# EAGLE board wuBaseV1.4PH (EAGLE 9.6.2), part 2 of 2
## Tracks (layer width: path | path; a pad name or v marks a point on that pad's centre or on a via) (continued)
GND  (via drill 0.35, 0.5) (continued)
  Bottom 0.508: R108.2 77.28,29.32 78.26,28.34 79,28.34 v79.86,29.2 | v90.8,32.74 90.36,32.29 89.83,32.29 89.64,32.48 C108.2 | v84.13,18.95 83.82,18.64 C66.2 | v83.31,17.47 83.31,17.7 83.3,17.71 C66.2 | C67.2 82.25,20.04 83.3,18.98 C66.2 | C59.2 77.03,16.99 77.16,17.12 v77.29,17.12 | C35.2 98.76,25.37 v98.5,25.62 | C119.2 87.34,23.29 88.28,24.23 v89.05,24.23 | 91.9,18.77 91.95,18.82 J1.1 | 105.1,25.62 C111.1 105.24,26.02 106,26.77 106.5,26.77 | 104.34,26.52 v104.34,27.78 | 101.7,23.47 102.05,23.81 | v92.84,17.39 92.76,17.39 | 103.33,24.1 C50.2 103.2,24.36 102.3,24.36 C51.2 | 102.39,23.76 102.44,23.81 | v103.4,22.83 103.45,22.78 104.78,22.78 v104.83,22.83 | C49.2 50.79,34.37 v52.53,33.24
  Bottom 0.61: C130.2 88.39,24.75 88.92,24.23 v89.05,24.23 | 91.9,18.77 91.01,18.77 v90.73,18.49 | v93.19,28.32 93.19,27.55 91.69,26.06 91.69,24.05 92.46,23.29 92.46,22.18 | 92.46,22.18 92.46,21.49 91.95,20.98 J1.1 91.95,18.21 92.76,17.39 | C50.2 103.97,24.49 105.1,25.62 | 101.83,23.47 100.89,22.53 v100.46,22.96 100.46,22.43 98.67,22.43 | C51.2 102.05,23.81 102.44,23.81 103.04,23.81 | J1.4 93.22,17.02 v92.84,17.39 | v104.83,22.83 105.24,23.25 C111.1 | 103.04,23.81 102.72,23.5 103.33,22.89 103.33,24.1 103.04,23.81 | 102.39,23.76 v102.39,22.86 102.39,22.98 101.91,23.47 101.83,23.47 | 101.83,23.47 101.7,23.47 | C3.1 v36.82,19.26 | C37.1 40.26,15.96 | 92.46,22.18 97.14,22.18
  Bottom 0.813: C111.1 104.34,26.52 | C21.1 37.45,19.77 37.07,21.16 36.44,21.8 v34.28,22.18
  Bottom 1.016: v36.82,19.26 37.45,19.77
  Bottom 1.27: 37.45,19.77 38.11,19.13 | 44.8,11.99 v45.09,10.79 v43.92,10.89 42.62,12.54
  Bottom 1.524: 38.11,19.13 40.26,15.96 42.62,12.54 44.8,11.99
  other vias: 83.2,28.67 85.11,28.67 87.02,28.67 85.11,30.2 85.11,27.28 72.34,33.88 110.08,25.65 90.27,34.52 78.44,32.48 79.71,32.48 80.98,32.48 79.83,23.47 78.82,23.21 101.55,27.78 102.95,26.39 80.67,24.33 98.96,31.34 107.64,33.88 53.92,33.75 71.7,34.64 80.21,16.99 87.83,12.92 109.57,20.19 73.74,12.92 91.67,21.33
  pour Bottom (isolate 0.203): 70.73,31.25 76.83,31.25 76.83,23.58 71.11,23.58 71.11,22.43 72.25,21.29 78.86,21.29 78.86,17.48 73.4,17.48 71.21,15.32 71.21,11.49 74.28,10.98 108.22,10.98 111.19,13.95 111.19,32.92 108.14,35.95 74.23,35.95 70.73,35.31
  pour Route2: 71.21,14.84 59.91,14.84 56.86,14.07 47.58,12.67 44.15,13.05 42.88,13.69 40.72,18.26 36.82,22.05 35.17,22.43 35.17,25.86 34.79,26.75 32.88,27.13 31.61,30.18 30.34,30.18 30.34,27.64 30.85,27.64 33.39,25.1 33.39,21.8 30.85,19.26 27.55,19.26 25.01,21.8 25.01,25.1 26.63,26.7 25.01,28.35 23.36,26.75 23.36,21.67 24.12,19.77 25.64,18.24 27.68,17.23 30.85,16.34 38.22,16.34 42.03,11.13 44.15,9.6 59.21,13.26 61.27,13.18 71.21,11.49
  pour Route2: 69.43,23.58 76.83,23.58 76.83,31.25 70.73,31.25 70.73,33.36 64.76,33.36 59.3,32.47 53.08,32.47 52.06,33.1 52.06,34.12 54.47,34.75 59.3,33.61 61.2,33.61 74.26,35.95 108.19,35.95 111.19,32.92 111.19,13.95 108.22,10.98 74.23,10.98 71.21,11.49 71.21,19.77 69.43,22.7
  pour Route15: 48.21,35.15 48.21,33.88 48.5,33.61 51.51,33.5 52.53,32.74 52.78,33.75 51.55,34.5 49.27,35.39 48.46,35.4
  cutout Bottom: 94.95,33.24 96.72,33.24 96.72,32.1 94.95,32.1
  pour Route15 (no thermals): 30.85,19.26 27.55,19.26 25.01,21.8 25.01,25.1 26.63,26.7 23.23,30.05 22.6,29.93 20.95,28.4 19.93,26.24 19.93,22.56 20.31,21.93 20.82,21.67 21.2,21.67 21.2,26.12 21.45,26.12 21.45,21.67 21.71,21.67 21.71,26.24 21.96,26.24 21.96,21.67 22.21,21.67 22.21,26.24 22.47,26.24 22.47,21.67 22.72,21.67 22.72,26.24 22.98,26.24 22.98,21.67 23.23,21.67 23.23,26.12 23.48,26.12 23.48,21.42 24.12,19.77 25.64,18.24 27.68,17.23 30.85,16.34 34.79,16.34 37.68,18.4 39.23,20.66 39.23,22.59 39.87,23.83 39.87,24.21 39.49,24.59 37.02,25.23 36.57,25.74 35.93,29.8 35.68,31.83 35.68,32.59 35.55,32.98 35.3,33.23 33.9,33.74 32.63,34.5 31.23,34.88 26.02,34.88 25.39,34.5 25.39,34.37 30.98,34.37 30.98,34.12 25.06,34.12 24.88,33.74 24.88,31.58 26.15,31.58 26.15,32.21 25.26,32.21 25.26,32.47 26.15,32.47 26.15,33.23 25.39,33.23 25.39,33.48 31.87,33.48 31.87,33.23 30.22,33.23 30.22,32.47 32.25,32.47 32.25,32.21 30.85,32.21 30.85,31.58 32.25,31.58 32.25,31.32 30.85,31.32 30.85,30.69 32.25,30.69 32.25,30.43 30.22,30.43 30.22,29.67 31.87,29.67 31.87,29.42 25.39,29.42 25.39,29.67 26.15,29.67 26.15,30.43 25.26,30.43 25.26,30.69 26.15,30.69 26.15,31.32 24.88,31.32 24.88,29.04 25.14,28.78 30.22,28.78 30.22,28.53 25.39,28.53 26.28,27.64 30.85,27.64 33.39,25.1 33.39,21.8
  pour Top: 64.76,33.36 72.63,33.36 72.63,35.64 61.2,33.61 59.3,33.61 54.47,34.75 52.06,34.12 52.06,33.1 53.08,32.47 59.3,32.47
  cutout Bottom: 88,23.45 88,21.93 88.64,21.93 88.64,23.45
  cutout Bottom: 69.84,26.88 70.47,26.88 70.47,25.86 69.84,25.86 69.84,26.75
HVMON_A
  Bottom 0.305: R32.1 R31.2 C36.1
HVMON_B  (via drill 0.35)
  Top 0.203: v56.59,19.66 56.08,19.66 55.32,20.29 v54.69,21.69 | v95.84,24.23 94.69,24.23 93.42,22.96 91.36,22.96 90.42,22.02 87.4,22.02 v86.84,21.46
  Route15 0.203: v56.59,19.66 56.72,19.78 63.07,19.78 64.34,21.05 69.55,21.05 69.78,21.28 86.67,21.28 v86.84,21.46
  Bottom 0.203: v95.84,24.23 96.27,24.66 99.95,24.66 100.17,24.88 C35.1 100.17,25.95 101.37,27.15 101.93,27.15 R30.2
  Bottom 0.254: R31.1 54.47,22.43 v54.69,21.69
K
  Top 0.508: R29.2 35.42,5.92 K.P$1
  Bottom 0.508: C48.2 34.03,8.59 K.P$1
  pour Route15 (no thermals): 32.38,9.73 33.14,10.24 34.15,10.11 35.55,9.35 36.69,7.45 36.82,6.43 35.68,4.91 35.04,4.91 33.14,7.96 32.38,8.21
K-DY1-AA  (via drill 0.35)
  Top 0.305: D14.2 v29.84,6.56 | R28.1 v29.84,6.56 | D13.1 v29.84,6.56
  Bottom 0.305: R14.2 C32.2 v29.84,6.56 C33.1 R15.1
  pour Route15: 27.47,5.52 28.44,6.2 28.49,7.35 30.9,7.73 31.36,7.07 31.33,5.67 32.02,5.21 32.1,5.01 32.1,4.15 31.61,1.94 30.72,0.97 27.68,0.97 26.91,1.35 26.71,2.01 26.71,3.28 27.45,4.45
K-DY1-AB  (via drill 0.35)
  Top 0.305: v29.84,9.1 R28.2
  Bottom 0.305: C47.2 v29.84,9.1 C48.1
  pour Route15: 28.18,9.23 28.18,7.96 28.34,7.78 31.28,8.16 31.54,8.36 31.51,9.76 31.08,10.14 28.59,9.81
K-DY1-BA  (via drill 0.35)
  Top 0.305: D12.1 v25.39,6.69 | D13.2 v25.39,6.69 | R27.1 v25.39,6.69
  Bottom 0.305: C31.2 R13.2 v25.39,6.69 C32.1 R14.1
  pour Route15: 27.17,7.45 25.26,7.83 23.74,9.1 23.36,9.1 23.1,8.84 23.1,7.7 22.34,7.09 22.09,6.71 22.09,5.92 22.37,5.04 22.37,3.64 22.6,2.24 23.61,1.22 24.88,1.1 25.64,1.35 25.85,1.86 25.85,3.51 26.66,4.65 26.66,5.67 27.42,6.3 27.42,7.07
K-DY1-BB  (via drill 0.35)
  Top 0.305: v26.02,9.23 R27.2
  Bottom 0.305: C46.2 v26.02,9.23 C47.1
  pour Route15: 22.49,9.63 22.47,10.75 22.85,11.13 23.87,10.88 25.39,10.11 26.79,9.86 27.17,9.61 27.42,9.23 27.42,8.21 27.17,7.96 25.39,8.21 23.74,9.48 23.26,9.38 22.85,9.35
KA  (via drill 0.35)
  Top 0.305: D14.1 v34.15,4.53 R29.1
  Bottom 0.305: v34.15,4.53 R15.2 C33.2
  pour Route15 (no thermals): 32.17,6.3 32.3,5.95 33.01,5.54 33.01,3.13 33.26,2.88 33.77,2.88 34.28,3.26 34.79,4.53 32.88,7.57 32.38,7.57 32.17,7.07
N$11
  Bottom 0.254: IC7.2 60.41,22.58 60.15,22.31 C79.2 59.77,22.2 R78.2
N$15
  Bottom 0.254: IC7.3 60.41,23.08 60.15,23.35 C83.1 59.77,23.47 R84.2
N$16
  Bottom 0.203: R87.2 56.88,24.23
  Bottom 0.254: R86.1 R84.1 57.77,23.34 56.88,23.34 | 56.88,23.34 C81.2 56.08,23.33 R83.2 | 56.88,24.23 56.88,23.34
N$17
  Bottom 0.254: R71.1 R78.1 57.77,22.32 56.88,22.32 | C81.1 56.88,22.32 | R77.2 56.85,22.29 56.88,22.32
N$18
  Bottom 0.254: IC7.1 60.42,21.34 C79.1 59.64,21.31 59.25,20.93 R71.2
N$19
  Bottom 0.254: IC7.4 60.39,24.35 C83.2 59.64,24.35 59.25,24.74 R86.2
N$22
  Bottom 0.203: R79.1 65.74,24.65 65.74,23.59 64.72,22.58
  Bottom 0.254: IC7.11 64.72,22.58
N$23
  Bottom 0.203: R85.1 65.23,26.68 65.23,23.84 64.47,23.08
  Bottom 0.254: IC7.10 64.47,23.08
N$25
  Bottom 0.254: IC6.2 58.61,28.66 C75.2 57.35,28.67 56.46,28.67 R69.2
N$26
  Bottom 0.254: IC6.3 58.05,29.18 57.66,29.57 57.48,29.57 C80.1 57.21,29.84 56.56,29.84 R73.2
N$27
  Bottom 0.254: R67.1 R69.1 55.23,28.93 54.34,28.93 C76.1 R68.2
N$28
  Bottom 0.254: R81.1 R73.1 55.23,29.94 54.34,29.94 C76.2 R72.2 53.8,30.84 53.43,31.2 R80.2
N$29
  Bottom 0.254: IC6.1 58.37,28.18 57.86,27.66 C75.1 57.18,27.66 57.12,27.59 57.06,27.53 R67.2
N$30
  Bottom 0.254: IC6.4 58.34,29.68 58.24,29.78 58.24,30.18 57.73,30.7 C80.2 57.06,30.7 56.45,31.34 R81.2
N$33
  Bottom 0.254: IC6.11 62.44,28.68 62.56,28.8 R70.1
N$34
  Bottom 0.254: IC6.10 61.92,29.18 62.7,29.95 R74.1
NRST
  Top 0.254: IC8.7 107.14,28.03 107.7,27.48 C94.1
REFH  (via drill 0.35)
  Top 0.254: IC10.9 67.21,27.15 66.66,26.61 | 66.66,26.61 C98.2 66.59,26.64 C101.1 | IC10.7 67.91,28.15 v67.77,28.29 | v67.26,25.88 67.26,26.01 66.66,26.61
  Route15 0.254: v67.77,28.29 67.13,27.66 67.13,26.01 v67.26,25.88
REFL  (via drill 0.35)
  Top 0.254: IC10.8 67.17,27.65 C98.1 | IC10.10 67.91,26.65 v67.77,26.51 | v67.26,28.93 66.62,28.29 C98.1 | C97.1 66.46,28.04 C98.1
  Route2 0.254: v67.77,26.51 67.13,27.15 67.13,28.8 v67.26,28.93
SPI1_MISO  (via drill 0.35)
  Top 0.203: IC8.32 99.49,27.01 98.31,27.01 v98.22,26.92 | v71.09,32.94 70.72,32.57 IC10.61 | v93.8,25.27 93.8,24.99 93.12,24.3 90.68,24.3 89.61,23.24 86.28,23.24 84.99,21.94 v83.9,21.94
  Route15 0.203: v73.48,21.81 73.66,21.64 83.59,21.64 v83.9,21.94 | v72.47,22.17 v72.47,22.18 72.47,29.18 71.09,30.55 v71.09,32.94
  Bottom 0.203: v73.48,21.81 73.38,21.71 72.83,21.71 72.47,22.07 v72.47,22.17 | v98.22,26.92 95.07,26.92 94.45,26.29 R89.2 93.83,25.24 v93.8,25.27
SPI1_MOSI
  Top 0.203: IC8.33 98.88,26.53 98.75,26.41 96.11,26.41 95.07,25.37 94.77,25.37 93.24,23.85 90.87,23.85 89.84,22.81 86.6,22.81 84.92,21.13 72.78,21.13 71.72,22.18 IC10.22
SPI1_SCK
  Top 0.203: IC8.39 101.2,23.75 101.04,23.59 99.9,23.59 99.19,24.3 96.52,24.3 96.09,24.74 94.69,24.74 93.37,23.41 91.14,23.41 90.1,22.38 86.93,22.38 85.3,20.75 72.42,20.75 71.22,21.94 IC10.21
SPI2_MISO
  Top 0.152: IC9.14 89.39,26.42 89.68,26.13 93.5,26.13 96.9,29.53 IC8.27
SPI2_MOSI  (via drill 0.35)
  Top 0.152: IC9.17 89.67,27.92 90.32,27.28 93.04,27.28 94.82,29.05 v94.82,29.31
  Top 0.203: IC8.28 v97.08,29.03
  Bottom 0.152: v94.82,29.31 95.2,28.93 96.98,28.93 v97.08,29.03
SPI2_SCK
  Top 0.152: IC9.15 89.53,26.92 89.94,26.51 93.37,26.51 96.89,30.03 IC8.26
SYNC  (via drill 0.35)
  Top 0.203: v93.16,29.18 92.9,28.92 IC9.19
  Route15 0.203: v93.16,29.18 92.91,28.93 92.35,28.93 91.05,27.63 91.05,19.08 91.39,18.74 91.39,18.26 90.88,17.75 v90.88,16.68
  Bottom 0.203: J1.8 95.76,14.63 95.19,14.07 91.39,14.07 91.01,14.45 91.01,16.56 v90.88,16.68
TIM2_CH3
  Top 0.203: IC8.12 106.72,30.53 107.02,30.83 107.02,31.09 107.53,31.59 R92.2
TIM2_CH3_SOFT  (via drill 0.35)
  Top 0.203: v46.28,11.76 49.01,11.51 59.97,14.05 70.6,14.05 72,12.65 v72.38,12.65 | v109.84,24.59 109.46,24.97 109.46,28.4 109.59,28.53 109.58,31.31 109.3,31.59 R92.1
  Top 0.305: IC1.3 36.2,19.91 v36.44,20.15
  Route15 0.203: v46.28,11.76 45.39,11.96 42.67,12.52 37.58,19.89 v36.44,20.15 | v72.38,12.65 72.96,12.07 104.82,12.07 108.32,15.58 108.32,20.4 109.84,21.93 v109.84,24.59
TRIGOUT  (via drill 0.35)
  Top 0.203: IC8.15 104.7,32.26 v104.6,32.36
  Top 0.254: v96.22,17.75 96.22,17.6 96.03,17.41 IC13.1 | v94.54,17.75 94.54,17.6 94.73,17.41 IC13.3
  Route15 0.152: v104.6,32.36 104.6,29.94 104.34,29.69 99.9,29.69 98.93,28.72 98.43,28.72 96.88,27.17 96.88,24.73 v97.83,23.78 | v94.54,17.75 94.54,17.98 95.07,18.51 95.84,18.51 96.22,18.13 v96.22,17.75
  Bottom 0.152: v97.83,23.78 97.73,23.68 97.73,21.8 97.22,21.29 96.64,21.29 96.38,21.04 96.38,17.92 v96.22,17.75
TRIGOUT_N  (via drill 0.35)
  Top 0.203: v93.83,18 93.8,18 93.45,17.65 93.45,16.89 93.11,16.55 R33.1
  Bottom 0.254: J1.5 94.31,19.54 94.31,18.49 v93.83,18
TRIGOUT_NA
  Top 0.203: IC13.4 93.42,14.81 R33.2 C123.1
TRIGOUT_P  (via drill 0.35)
  Top 0.203: R34.1 98.14,17 v98.5,17.37
  Route15 0.152: v94.03,17.17 94.11,17.24 98.38,17.24 v98.5,17.37
  Bottom 0.254: J1.6 94.41,15.73 94.41,16.79 v94.03,17.17
TRIGOUT_PA
  Top 0.203: R34.2 97.14,15.03 C124.1 96.2,14.98 IC13.6
TVS_OUT
  Top 0.305: R2.2 D1.C
UART_RXD_P  (via drill 0.35)
  Route15 0.152: v98.05,27.61 97.23,26.79 97.23,25.29 98.53,24 v98.53,23.8
  Bottom 0.152: 97.66,17.32 97.66,21.16 98.02,21.51 98.02,23.29 v98.53,23.8
  Bottom 0.203: R90.1 98.85,28.41 v98.05,27.61
  Bottom 0.254: 97.66,17.32 98.3,16.68 J1.12
UART_TXD_A  (via drill 0.35)
  Top 0.152: 105.63,21.16 105.63,21.32 105.4,21.54 104.64,21.54 104.08,20.99 104.08,20.92 | 105.63,21.16 IC11.1 | R93.1 105.64,21.16 105.63,21.16 | 104.08,20.92 104.33,20.67 IC11.3 | v96.77,22.95 97.08,22.64 98.16,22.64 101.84,21.54 103.46,21.54 104.08,20.92
  Top 0.203: R91.1 97.01,27.02 95.96,27.02 v95.33,26.39
  Route15 0.152: v96.77,22.95 96.77,22.98 96.26,23.48 95.84,23.48 95.33,24 v95.33,26.39
UART_TXD_N  (via drill 0.35)
  Top 0.203: v101.12,18.11 101.76,18.11 R99.1
  Bottom 0.254: J1.15 100.84,18.39 v101.12,18.11
UART_TXD_NA
  Top 0.203: IC11.4 102.95,17.92 R99.2 C112.1
UART_TXD_P  (via drill 0.35)
  Top 0.203: R98.1 100.08,16.95 v100.08,17.45
  Bottom 0.254: J1.14 99.57,16.81 100.08,17.32 v100.08,17.45
UART_TXD_PA  (via drill 0.35)
  Top 0.203: v103.02,15.77 102.84,15.59 102.43,15.59 R98.2 | IC11.6 105.73,17.81 v106.36,17.81 107.18,17.81 C113.1
  Route15 0.203: v103.02,15.77 105.06,17.8 v106.35,17.8 v106.36,17.81
USART1_RX  (via drill 0.35)
  Top 0.152: IC8.31 98.76,27.53 v98.73,27.55
  Bottom 0.203: R90.2 98.88,27.41 v98.73,27.55
USART1_TX
  Top 0.152: IC8.30 98.89,28.03 98.76,28.16 97.19,28.16 R91.2
VCCPLL  (via drill 0.5)
  Top 0.203: IC9.29 85.86,32.47 86.13,32.74 86.13,33.17 v86.23,33.27
  Top 0.508: v90.8,33.7 90.86,33.64 91.8,33.64 C109.1
  Bottom 0.508: v86.23,33.27 86.64,32.86 R94.2 87.67,32.86 C108.1 88.04,33 88.31,33.27 90.06,33.27 90.5,33.7 v90.8,33.7
VDD_AMP  (via drill 0.5)
  Top 0.305: L17.1 69.41,19.78 L16.1 72.24,19.27 73.14,18.37 74.79,18.37 76.04,19.61 88.41,19.61 89.87,18.16
  Top 0.508: v97.03,18.03 97.03,18.72 C115.1 92.44,18.75 91.3,17.61 90.41,17.61 89.87,18.16
  Bottom 0.508: J1.9 v97.03,18.03
VDDA-ADC  (via drill 0.5)
  Top 0.203: IC10.17 69.22,22.89 69.04,22.7
  Top 0.254: IC10.63 69.72,32.12 69.59,32.25 | IC10.64 69.22,32.17 69.14,32.25 | 68.38,32.25 v68.28,32.36 | IC10.1 68.21,31.15 68.1,31.26 | IC10.16 68.41,23.65 68.29,23.53 68.21,23.53
  Top 0.508: 68.21,23.53 v67.66,22.98 67.78,22.98 68.06,22.7 69.04,22.7 | 68.38,32.25 69.14,32.25 69.59,32.25 | 68.1,31.26 68.1,32.18 v68.28,32.36
  Bottom 0.406: v68.28,32.36 68.54,32.09 C91.1 68.54,30.06 69.38,29.22 C128.2 69.55,26.21 L18.2 69.55,24.58 68.78,23.81 C103.1
  Bottom 0.508: v67.66,22.98 68.27,23.59 C103.1
VDDFPGA  (via drill 0.5)
  Top 0.508: C114.1 97.97,21.4 97.93,21.36 v95.71,21.36 95.71,20.93 L19.1
  Bottom 0.508: v95.71,21.36 95.76,21.31 J1.7
VDDFPGA-FILT  (via drill 0.5)
  Top 0.203: v84.36,24.24 v84.35,24.23 | IC9.30 85.36,32.87 v85.31,32.91
  Top 0.229: IC9.5 v84.36,24.24
  Top 0.508: L19.2 93.81,20.16 93.1,19.45 90.5,19.45 v90.37,19.33
  Route15 0.406: v84.35,24.23 85.62,24.23 86.39,23.47 88.6,23.47 90.37,21.69 v90.37,19.33
  Route15 0.61: v91.46,31.21 91.08,31.21 89.81,32.48 88.82,32.48 88.61,32.28 85.95,32.28 v85.31,32.91
  Bottom 0.508: C107.1 85.11,32.71 v85.31,32.91 86.37,31.86 R94.1
  Bottom 0.61: v91.46,31.21 91.59,31.09 91.59,29.31 88.63,26.36 C130.1 87.29,26.36 85.55,24.61 C100.1 84.73,24.61 v84.35,24.23
VDDSW  (via drill 0.5)
  Top 0.508: C122.1 96.97,12.8 v95.94,12.8
  Route15 0.508: v94.56,33.88 97.11,33.88 97.87,34.64 108.15,34.64 109.98,32.81 109.98,26.95 109.04,26.01 109.04,22.32 v108.53,21.81
  Bottom 0.406: IC12.4 94.66,33.79 v94.56,33.88 94.56,32.48 94.32,32.24 | C132.2 R101.2 94.32,32.24 | 94.32,32.24 94.53,32.24 IC12.3
  Bottom 0.508: J1.10 97.03,13.61 96.22,12.8 v95.94,12.8 104.65,12.8 107.69,15.83 107.69,20.91 108.53,21.76 v108.53,21.81
VDDSW-FILT  (via drill 0.35, 0.5)
  Top 0.305: v45.92,12.37 49.12,12.09 59.97,14.45 75.19,14.45 76.95,16.21 82.03,16.21 v82.54,16.72
  Top 0.508: v92.41,29.69 92.41,29.75 93.42,30.77 L13.2
  Route15 0.305: v89.36,21.05 88.8,20.49 84.58,20.49 82.54,18.46 v82.54,16.72 | v45.92,12.37 45.42,12.37 42.95,12.87 37.81,20.45 v35.8,20.91
  Bottom 0.406: C119.1 89.36,22.69 v89.36,21.05 | v35.8,20.91 35.41,20.91 R1.1
  Bottom 0.508: C119.1 90.25,23.61 90.25,26.89 92.41,29.05 v92.41,29.69
VDDSW-FILT-RL
  Bottom 0.406: R1.2 33.02,20.48 31.85,19.31 L1.2
VDDSW-FINAL  (via drill 0.35)
  Top 0.406: v32.63,18.57 32.63,18.36 32.73,18.26 32.73,17.88 C1.2 | IC1.6 33.03,18.21 32.65,18.13 C1.2 | C2.2 C1.2
  Bottom 0.406: L1.1 32.85,18.14 32.63,18.36 v32.63,18.57
VDDSW-RL  (via drill 0.5)
  Top 0.508: L13.1 94.12,32.67 93.55,33.24 v93.55,34.01
  Bottom 0.305: IC12.5 95.84,34.26 95.45,34.64 94.18,34.64 v93.55,34.01 93.55,33.36 R101.1
VDDSW_IMON  (via drill 0.35)
  Top 0.203: R111.2 v101.17,33.88
  Bottom 0.203: v101.17,33.88 100.52,33.23 97.04,33.23 IC12.6
VDDU  (via drill 0.5)
  Top 0.508: C127.1 101.06,14.19 v100.86,13.99
  Route15 0.508: v100.86,13.99 99.06,13.99 97.73,15.32 87.34,15.32 v86.83,14.81
  Bottom 0.305: L18.1 70.61,24.55 70.61,22.44 71.8,21.26 82.96,21.26 84.8,19.41 84.8,16.72 86.71,14.81 v86.83,14.81
  Bottom 0.508: v100.86,13.99 100.84,14.02 J1.16 100.93,15.65 109.03,23.75 L15.1 L11.1
VDDU-FILT  (via drill 0.35, 0.4, 0.45, 0.5)
  Top 0.203: IC9.33 83.86,32.84 v83.84,32.86 | IC9.24 89.13,31.42 v89.3,31.59 | 89.35,30.42 | IC9.1 82.36,25.12 82.21,24.97
  Top 0.229: IC9.22 89.35,30.42
  Top 0.254: IC10.42 77.94,28.15 78.31,28.52 78.31,28.6 | 78.47,28.76 C105.1 | IC8.48 105.7,24.22 106.5,23.42 C85.1 | IC8.24 100.2,31.73 99.71,32.21 C99.1 | IC8.36 99.39,25.03 99.26,24.91 | IC8.1 106.51,25.03 106.86,24.68 v106.86,23.8
  Top 0.305: R104.2 97.34,31.62 v97.46,31.62 | R93.2 107.49,23.16 v106.86,23.8 | IC1.5 v32.7,19.26
  Top 0.406: C105.1 78.61,28.75 v78.61,29.56 | 89.35,30.42 89.91,30.42 v90.06,30.58 | v106.86,23.8 106.85,23.8 106.49,23.44 C85.1 | C88.1 99.26,24.87 99.26,24.91 | C99.1 98.35,32.21 C121.2 98.12,32.28 v97.46,31.62 | IC11.5 104.98,16.81 C118.1 105.04,16.76 v106.12,16.76 | C133.1 95.2,13.6 95.33,13.73 | 95.33,13.73 95.93,13.73 v95.94,13.74 | IC13.5 95.38,13.77 95.33,13.73 | IC1.1 36.07,18.61 v36.44,18.24 | IC4.5 88.19,18.91 88.89,18.21 88.89,16.51 C64.2 88.9,14.22 89.35,13.76 v89.69,13.76
  Top 0.508: 78.31,28.6 78.47,28.76 | 82.21,24.97 81.58,24.97 v81.43,25.12 | C88.1 96.82,24.87 v96.14,25.55
  Route15 0.406: v36.44,18.24 37.18,18.34 37.86,18.7 42.34,12.11 45.63,11.46 46.22,10.95 46.95,10.95 59.3,13.8 89.65,13.8 v89.69,13.76
  Route15 0.508: v90.06,30.58 90.32,30.58 90.44,30.45 90.95,30.45 | 90.95,30.45 91.46,29.94 91.46,29.18 88.79,26.51 82.82,26.51 v81.43,25.12 | 96.14,29.56 96.47,29.56 97.23,30.32 97.23,31.39 v97.46,31.62 98.96,33.12 v108.41,33.12 109.27,32.25 109.27,27.25 106.86,24.84 v106.86,23.8 107.19,23.47 107.19,17.57 106.38,16.76 v106.12,16.76 105.26,16.76 101.55,13.05 97.11,13.05 96.42,13.74 v95.94,13.74 95.76,13.74 95.51,13.48 89.97,13.48 v89.69,13.76 | 96.14,29.56 95.58,29.56 94.69,30.45 90.95,30.45 | v96.14,25.55 96.14,29.56
  Route15 0.813: v78.61,29.56 79.5,30.45 81.43,30.45 v83.84,32.86 85.36,31.34 89.05,31.34 v89.3,31.59 89.3,31.34 v90.06,30.58
  Bottom 0.305: v108.41,33.12 108.92,32.6 R64.1 | R89.1 95.65,25.45 96.04,25.45 v96.14,25.55 | v32.7,19.26 33.77,19.26 34.78,18.25 C3.2
  Bottom 0.508: v83.84,32.86 C104.1 | v90.06,30.58 89.55,30.06 C106.1 | C96.1 81.81,25.5 v81.43,25.12 | v89.3,31.59 88.41,30.7 C110.1 | L15.2 107.39,24.48 106.86,23.95 v106.86,23.8 | C3.2 v36.44,18.24
VDDUA  (via drill 0.5)
  Top 0.254: IC8.9 107.39,29.03 107.94,29.61 C93.1
  Top 0.305: v107.65,30.58 107.65,30.45 108.01,30.09 C93.1
  Bottom 0.203: R16.1 105.23,31.33 106.8,32.91 R35.1 107.6,32.91 108.03,32.48 108.03,30.96 v107.65,30.58
  Bottom 0.406: v107.65,30.58 107.65,30.45 108.79,29.31 108.79,27.02 108.03,26.27 L11.2 106.97,25.75 C111.2
VREF  (via drill 0.35)
  Top 0.203: v64.34,32.1 64.34,32.61 64.62,32.89 66.11,32.89 66.9,32.1 C95.1 67.81,32.99 69.72,32.99 70.22,32.49 IC10.62
  Top 0.254: L9.1 63.82,32.23 64.21,32.23 v64.34,32.1
  Bottom 0.254: v64.34,32.1 64.34,30.63 64.92,30.04 64.92,28.75 64.29,28.11 63.65,28.11 62.64,27.1 62.38,27.1 61.01,25.74 59.27,25.74 58.75,26.26 L10.1
VREF_FILT1
  Bottom 0.254: L10.2 56.22,26.39 53.85,26.39 53.51,26.04 C84.1 54.47,24.47 R83.1
VREF_FILT2  (via drill 0.3)
  Top 0.254: L9.2 62.19,31.85 60.96,31.85 60.37,31.25 C78.1 59.64,31 58.72,31 v58.55,30.83
  Bottom 0.254: R72.1 54.57,32.1 57.28,32.1 v58.55,30.83
VSS_AMP  (via drill 0.5)
  Top 0.508: C116.1 99.31,18.6 v99.31,17.93
  Route15 0.508: v74.88,15.46 75.13,15.46 75.64,15.97 98.22,15.97 99.31,17.06 v99.31,17.93
  Bottom 0.305: v74.88,15.46 74.85,15.5 L14.1 73.54,15.5 72.74,16.3 L12.1
  Bottom 0.508: J1.13 99.57,18.18 v99.31,17.93

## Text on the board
tPlace: wuBaseV1.4PH / WIPAC 2023
bPlace: BLK2 | BLK2 | BLK1 | BLK1
Measures: The outline in this layer is for LOM16 / with 55mm neck-diameter NNVT, but / no allowance added for HA coating, / according to design files 2021-11-22
Document: The outline in this layer is for LOM16 / with 55mm neck-diameter NNVT, plus / additional 1mm diameter for HA coating, / according to design files 2021-11-23
Reference: The outline in this layer is for LOM16 / with 55mm neck-diameter NNVT, plus / additional 1mm diameter for HA coating, / according to design files 2021-11-23 | N.B. the PMT pin circle diameter / is the one for NNVT PMT, 31.8mm. / The Hamamatsu circle is 34mm.
Mechanical: The outline in this layer is the common polar / outline proposal implemented in the file / wuBaseV1.4PH-work, 2023-02-16
Patch_Top: The outline in this layer is for LOM16 / with 55mm neck-diameter NNVT, plus / additional 1mm diameter for HA coating, / HV region expanded corresponding to / moving the PCB to 6mm distance from / PMT (previously 8mm). Design 2021-11-26.
Vscore: The outline in this layer is a repeat, / checking that it agrees with previous / version intended for LOM16 with 55mm / neck-diameter NNVT plus additional / 1mm diameter for HA coating. New / version is imported from Vedant's / design file 2021-11-30.
fp3: 2022-11-17: The outline in this layer / matches PSL LOM16 model. It is the same / as from 2021-11-30, but with "ears" added / for alignment. The original version was for / 54mm neck-diameter Hamamatsu, / plus additional 1mm diameter for HA / coating. Compared to the design before / that, this one had some expanded / area in critical HV regions, and a bit / narrower isthmus. The narrower isthmus / was chosen to give 5mm clearance to the / nearest neighbor, rather than 4.5mm as / in previous design.
Name: The outline in this layer is similar to the latest LOM 16 equatorial / outline (end of 2022) but with an additional cut near the ribbon / cable connector, that would allow it to also fit in the LOM 18 / (see Slack message from Nobu 2023-02-08), and then / I also adjusted other parts of the outline as a trial balloon / to see if the latest LOM16 and LOM18 arrangements / would be ok with such changes. Not intended to be final. 2023-02-16
fp9: The outline in this layer is the one from 2021-11-30, / which was given to PSL for LOM16 design, and then / it had "ears" added for orientation that are shown in / a different layer.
